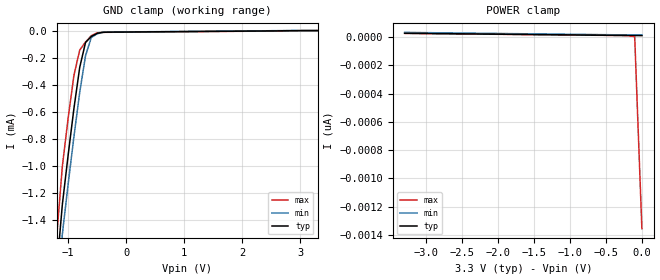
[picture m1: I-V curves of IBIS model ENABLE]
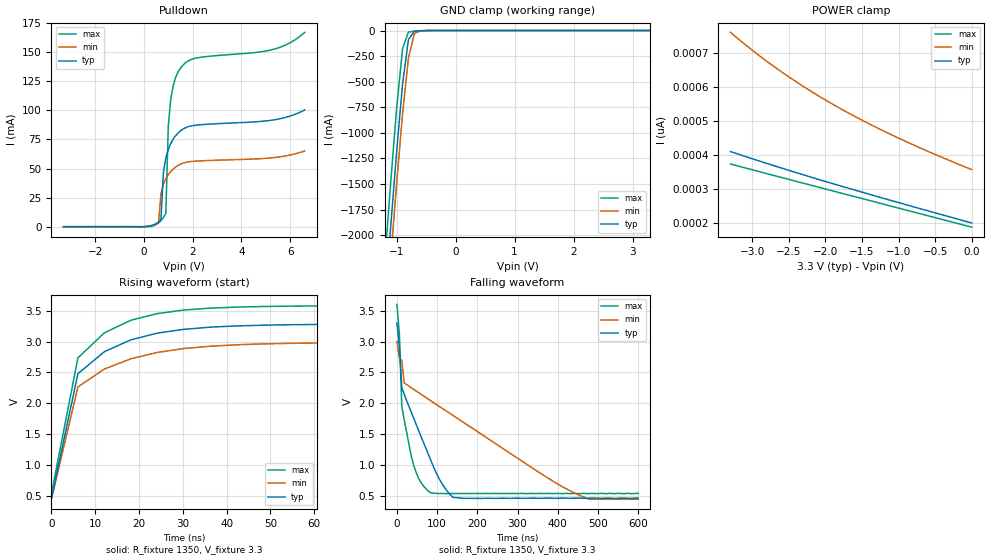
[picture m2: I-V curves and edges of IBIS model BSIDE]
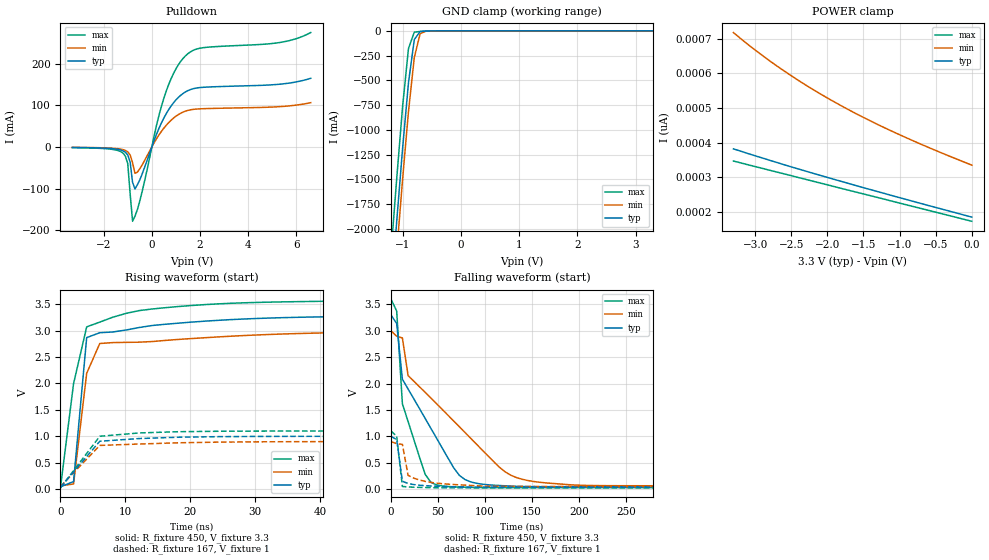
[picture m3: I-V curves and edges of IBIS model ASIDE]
| PCA9508 IBIS Model
[IBIS Ver]   4.0
[Comment Char]   |_char
| vdd: nom:3.3v, min:3v, max:3.6v
[File name]   pca9508.ibs
[File Rev]   2
[Date]   September 14, 2009 4:38:58 PM
[Source]
Generated by Nipun Chaplot at NXP Tempe using IBIS Toolkit
[Notes]
|The package model information is simulated at 400 kHz,
|which is the maximum system operating frequency.
[Disclaimer]
(C) Copyright 2007 NXP Semiconductors
All rights reserved
NXP Semiconductors (NXP) does not warrant that this model and any other
accompanying information (Model) accurately or fully represents the
operating characteristics and specifications of the semiconductor
products to which the Model relates.  Moreover, the Model is furnished
on an "as is" and with "all faults" basis, and without support or
warranty of any kind.  NXP disclaims all warranties, whether expressed
or implied or statutory, including without limitation all implied
warranties of non-infringement, merchantability and fitness for any
purpose, and those arising from a course of dealing or usage of trade.
NXP does not convey any license under its or any third party's patents,
copyrights or other intellectual property or proprietary rights.
You and your company assume any and all risks and liability arising out
of the application or use of the Model.
In no event shall NXP be liable for any direct, indirect, special,
consequential or incidental damages, however caused, whether in
warranty, contract or tort (including negligence), strict liability or
other legal theory, including, without limitation, for lost profits,
business interruption, or corruption or loss of data or information,
arising out of or in connection with the use of or the inability to use
the Model, even if NXP has been advised of the possibility of such
damages.
NXP provides the Model as a courtesy to our customers. You and your
company shall not distribute, convey, sell, or give the Model to anyone
else without receiving prior written permission from NXP.
NXP reserves the right to make changes without notice to the Model to
improve reliability, function, or design.
Please be aware that your receipt and subsequent use of the Model shall
serve as acceptance of these terms and conditions.  If you do not
accept these terms, return or destroy the Model immediately.
[Copyright]
(C) Copyright 2009 NXP Semiconductors  All rights reserved
| TSSOP8 Package
[Component]   PCA9508DP
Si_location Die
Timing_location Pin
[Manufacturer]   NXP Semiconductors
[Package]
|Simulation frequency: 100MHz
|variable   typ   min   max
R_pkg   33.7m   30.1m   37.3m
L_pkg   1.74n   1.67n   1.81n
C_pkg   0.428p   0.422p   0.434p
[Pin] signal_name   model_name   R_pin   L_pin   C_pin
1   VCCA   POWER   5.47E-02  2.21E-09  4.81E-13
2   SCLA   ASIDE   4.14E-02  1.54E-09  4.20E-13
3   SDAA   ASIDE   4.14E-02  1.55E-09  4.20E-13
4   GND   GND   5.47E-02  2.21E-09  4.80E-13
5   EN   ENABLE   5.47E-02  2.21E-09  4.78E-13
6   SDAB   BSIDE   4.14E-02  1.55E-09  4.17E-13
7   SCLB   BSIDE   4.14E-02  1.54E-09  4.17E-13
8   VCCB   POWER   5.47E-02  2.21E-09  4.79E-13
[Package Model]   tssop8_sot505EC12
|The package model information is simulated at 400 kHz,
|which is the maximum system operating frequency.
| SO-8 package
[Component]   PCA9508D
Si_location Die
Timing_location Pin
[Manufacturer]   NXP Semiconductors
[Package]
|Simulation frequency: 100MHz
|variable   typ   min   max
R_pkg   4.81E-02   4.14E-02   5.47E-02
L_pkg   1.88E-09   1.54E-09   2.21E-09
C_pkg   0.449E-12   0.417E-12   0.481E-12
[Pin] signal_name   model_name   R_pin   L_pin   C_pin
1   VCCA   POWER   37.3m   1.81nH   0.428pF
2   SCLA   ASIDE   30.1m   1.67nH   0.422pF
3   SDAA   ASIDE   30.1m   1.67nH   0.428pF
4   GND   GND   37.3m   1.81nH   0.434pF
5   EN   ENABLE   37.3m   1.81nH   0.428pF
6   SDAB   BSIDE   30.1m   1.67nH   0.422pF
7   SCLB   BSIDE   30.1m   1.67nH   0.428pF
8   VCCB   POWER   37.3m   1.81nH   0.434pF
[Package Model]   so8_sot96bl53
|   PACKAGE MODEL SO-8
[Define Package Model]  so8_sot96bl53
[Manufacturer]  NXP
[OEM]   NXP Semiconductors
[Description]   Full package IBIS model.Simulated @ 400kHz
[Number Of Pins]  8
[Pin Numbers]
|Pin Num   Terminal Name
1   | Lead1:pin1
2   | Lead2:pin2
3   | Lead3:pin3
4   | Lead4:pin4
5   | Lead5:pin5
6   | Lead6:pin6
7   | Lead7:pin7
8   | Lead8:pin8
[Model Data]
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[End Model Data]
[End Package Model]
|   PACKAGE MODEL TSSOP8
[Define Package Model]  tssop8_sot505EC12
[Manufacturer]  NXP
[OEM]   NXP Semiconductors
[Description]   Full package IBIS model. Simulated @ 400kHz
[Number Of Pins]  8
[Pin Numbers]
|Pin Num   Terminal Name
1   | Lead1:pin1
2   | Lead2:pin2
3   | Lead3:pin3
4   | Lead4:pin4
5   | Lead5:pin5
6   | Lead6:pin6
7   | Lead7:pin7
8   | Lead8:pin8
[Model Data]
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[End Model Data]
[End Package Model]
| Models and submodels in the file (3): ENABLE (Input), BSIDE (I/O_open_drain), ASIDE (I/O_open_drain)
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|The package model information is simulated at 400 kHz,
|which is the maximum system operating frequency.
[Model]   ENABLE
Model_type Input
Vinh=2.31
Vinl=0.99
|Subparameter   typ   min   max
C_comp   1.86p   1.7p   2p
[Model Spec]
Vinh   2.31   1.89   5.5
Vinl   0.99   0.40   1.65
[Temperature Range] 27   85   -40
[Voltage Range]   3.3   3   3.6
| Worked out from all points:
|   GND clamp passes 1 mA (typ) near -1.02 V on its own axis
[GND Clamp]
-3.3V     -17.95A    -17.36A    -18.67A
-1.2V     -1.789mA   -2.001mA   -1.542mA
-1.1V     -1.289mA   -1.508mA   -1.007mA
-1V       -922.8uA   -1.138mA   -649.1uA
-900mV    -576.7uA   -785.3uA   -331.4uA
-800mV    -272.4uA   -456.9uA   -144.1uA
-700mV    -88.06uA   -186.1uA   -84.85uA
-600mV    -43.6uA    -50.75uA   -37.68uA
-500mV    -20.3uA    -24.22uA   -16.64uA
-300mV    -11.67uA   -10.77uA   -12.63uA
3.3V      9.969pA    13.77pA    -1.356nA
[POWER Clamp]
-3.3V     26.62pA    32.76pA    25.82pA
-200mV    11.03pA    14.89pA    10.27pA
-100mV    10.53pA    14.32pA    2.629pA
0V        9.962pA    13.77pA    -1.356nA
[Model]   BSIDE
Model_type I/O_open_drain
Vinh=2.31
Vinl=0.99
Vref=3.3
Vmeas=0.65
Rref=1350
Cref=50p
|Subparameter   typ   min   max
C_comp   4.28p   4.1p   4.4p
[Model Spec]
Vinh   2.31   1.89   5.5
Vinl   0.99   0.40   1.65
Vmeas   1.65   1.35   2.75
[Temperature Range] 27   85   -40
[Voltage Range]   3.3   3   3.6
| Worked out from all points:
|   slope of the pulldown table from 0 to 0.495 V, typ, clamps not added: 200 ohm
|   GND clamp passes 1 mA (typ) near -0.52 V on its own axis
|   falling waveform, R_fixture 1350, V_fixture 3.3: 20-80 % time 79.4ns typ, 320ns min, 28.8ns max; typ from 3.3 V to 0.464 V
|   rising waveform, R_fixture 1350, V_fixture 3.3: 20-80 % time 8.61ns typ, 8.99ns min, 8.11ns max; typ from 0.463 V to 3.3 V
[Pulldown]
-3.3V     0A         0A         0A
600mV     3.943mA    3.455mA    3.206mA
700mV     6.084mA    27.99mA    5.214mA
800mV     46.34mA    36.75mA    7.871mA
900mV     59.04mA    41.34mA    11.66mA
1V        66.35mA    44.71mA    86.27mA
1.1V      71.51mA    47.35mA    109.2mA
1.3V      78.18mA    51.26mA    128.3mA
1.5V      82.38mA    53.79mA    136.3mA
2.2V      87.4mA     56.44mA    145.2mA
5.4V      92.07mA    59.57mA    153mA
6.6V      100.4mA    65.12mA    167.1mA
[GND Clamp]
-3.3V     -37.68A    -37.34A    -38.04A
-1.2V     -2.671A    -2.981A    -2.242A
-1.1V     -1.91A     -2.223A    -1.478A
-1V       -1.181A    -1.492A    -758.7mA
-900mV    -524.4mA   -815.2mA   -178.8mA
-800mV    -88.63mA   -269.5mA   -14.24mA
-700mV    -7.072mA   -29.66mA   -6.721mA
-600mV    -2.61mA    -3.048mA   -2.176mA
3.3V      200.1pA    356.8pA    187.8pA
[POWER Clamp]
-3.3V     410pA      760.5pA    373.4pA
-2.9V     381.9pA    691pA      350.8pA
-2.6V     361.6pA    644.2pA    333.8pA
-2.2V     335pA      587.6pA    311.2pA
-1.8V     309.4pA    536.8pA    288.7pA
-1.3V     278.3pA    480.4pA    260.7pA
-900mV    253.9pA    439.5pA    238.2pA
0V        200.1pA    356.8pA    187.8pA
[Falling Waveform]
R_fixture=1350
V_fixture=3.3
V_fixture_min=3
V_fixture_max=3.6
0s        3.3V       3V         3.6V
6.061ns   2.917V     2.739V     3.13V
12.12ns   2.252V     2.693V     1.951V
18.18ns   2.149V     2.326V     1.729V
42.42ns   1.749V     2.222V     978.8mV
78.79ns   1.165V     2.064V     571.2mV
109.1ns   731.6mV    1.933V     538.9mV
139.4ns   475.2mV    1.803V     538.5mV
454.5ns   463.7mV    508.8mV    537.1mV
600ns     464.1mV    448mV      540.8mV
[Rising Waveform]
R_fixture=1350
V_fixture=3.3
V_fixture_min=3
V_fixture_max=3.6
0s        462.9mV    449.4mV    539.4mV
6.061ns   2.482V     2.267V     2.737V
12.12ns   2.837V     2.557V     3.143V
18.18ns   3.029V     2.722V     3.345V
24.24ns   3.137V     2.825V     3.453V
30.3ns    3.198V     2.888V     3.51V
36.36ns   3.233V     2.925V     3.541V
48.48ns   3.265V     2.962V     3.567V
84.85ns   3.284V     2.986V     3.582V
600ns     3.299V     2.998V     3.599V
[Ramp]
R_load=1350
dV/dt_r   4.966E-3/1.215E-8   2.879E-3/1.635E-8   7.929E-3/7.340E-9
dV/dt_f   1.702E+0/7.706E-8   1.531E+0/3.202E-7   1.836E+0/2.904E-8
|[End   BSIDE
[Model]   ASIDE
Model_type I/O_open_drain
Vinh=2.31
Vinl=0.99
Vref=3.3
Vmeas=0.65
Rref=450
Cref=50p
|Subparameter   typ   min   max
C_comp   3.97p   3.8p   4.1p
[Model Spec]
Vinh   2.31   0.63   5.5
Vinl   0.99   0.27   1.65
Vmeas   0.99   0.27   1.65
[Temperature Range] 27   85   -40
[Voltage Range]   3.3   3   3.6
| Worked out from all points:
|   slope of the pulldown table from 0 to 0.495 V, typ, clamps not added: 7.18 ohm
|   GND clamp passes 1 mA (typ) near -0.52 V on its own axis
|   falling waveform, R_fixture 450, V_fixture 3.3: 20-80 % time 48.3ns typ, 86ns min, 20.1ns max; typ from 3.3 V to 0.044 V
|   falling waveform, R_fixture 167, V_fixture 1: 20-80 % time 4.46ns typ, 9.58ns min, 4.11ns max; typ from 1 V to 0.035 V
|   rising waveform, R_fixture 450, V_fixture 3.3: 20-80 % time 1.45ns typ, 2.27ns min, 2.95ns max; typ from 0.043 V to 3.3 V
|   rising waveform, R_fixture 167, V_fixture 1: 20-80 % time 4.03ns typ, 3.98ns min, 4.01ns max; typ from 0.035 V to 1 V
[Pulldown]
-3.3V     -1.37mA    -1.08mA    -1.78mA
-1.2V     -9.287mA   -6.495mA   -14.72mA
-1V       -19.25mA   -11.89mA   -40.21mA
-900mV    -36.58mA   -19.24mA   -112.9mA
-800mV    -85.08mA   -38.24mA   -178.8mA
-700mV    -101.1mA   -63.27mA   -166.5mA
-600mV    -91mA      -60.81mA   -150.6mA
500mV     69.44mA    45.13mA    117mA
900mV     106mA      69.26mA    176.4mA
1.4V      132.3mA    86.05mA    219mA
2V        142.6mA    91.51mA    237.3mA
6.6V      164.9mA    106.3mA    274.8mA
[GND Clamp]
-3.3V     -37.68A    -37.34A    -38.04A
-1.2V     -2.671A    -2.981A    -2.242A
-1.1V     -1.91A     -2.223A    -1.478A
-1V       -1.181A    -1.492A    -758.5mA
-900mV    -524.1mA   -815mA     -178.5mA
-800mV    -88.25mA   -269.1mA   -13.8mA
-700mV    -6.842mA   -29.34mA   -6.41mA
-600mV    -2.483mA   -2.935mA   -2.068mA
3.3V      185.4pA    335.3pA    173.4pA
[POWER Clamp]
-3.3V     382.2pA    717.4pA    347pA
-3V       362.2pA    667.1pA    331.2pA
-2.6V     336.6pA    607pA      310.2pA
-2.2V     312pA      553.4pA    289pA
-1.8V     288pA      505.5pA    267.9pA
-1.3V     258.8pA    452.1pA    241.7pA
-1V       241.5pA    422.9pA    225.8pA
-500mV    213.3pA    377.6pA    199.6pA
0V        185.4pA    335.3pA    173.4pA
[Falling Waveform]
R_fixture=450
V_fixture=3.3
V_fixture_min=3
V_fixture_max=3.6
0s        3.3V       3V         3.6V
6.061ns   3.137V     2.896V     3.374V
12.12ns   2.082V     2.864V     1.617V
18.18ns   1.896V     2.151V     1.28V
36.36ns   1.338V     1.832V     279.6mV
48.48ns   963.1mV    1.617V     77.99mV
78.79ns   179.2mV    1.071V     35.55mV
121.2ns   62.41mV    327.7mV    28.42mV
151.5ns   46.21mV    144.1mV    28.23mV
600ns     44.04mV    62.24mV    28.14mV
[Falling Waveform]
R_fixture=167
V_fixture=1
V_fixture_min=0.9
V_fixture_max=1.1
0s        1V         900mV      1.1V
6.061ns   936mV      860.2mV    1.003V
12.12ns   148.4mV    846.9mV    49.72mV
18.18ns   105.1mV    260.1mV    40.3mV
24.24ns   85.33mV    207.1mV    35.22mV
36.36ns   64.21mV    145.7mV    29.46mV
60.61ns   45.37mV    93.13mV    23.67mV
96.97ns   35.98mV    58.01mV    23.02mV
127.3ns   35.39mV    50.32mV    22.95mV
600ns     35.12mV    48.44mV    22.9mV
[Rising Waveform]
R_fixture=450
V_fixture=3.3
V_fixture_min=3
V_fixture_max=3.6
0s        43.1mV     61.36mV    27.03mV
2.02ns    142.9mV    96.25mV    1.996V
4.04ns    2.869V     2.192V     3.072V
6.061ns   2.961V     2.757V     3.162V
8.081ns   2.975V     2.774V     3.255V
12.12ns   3.06V      2.782V     3.38V
16.16ns   3.121V     2.815V     3.435V
26.26ns   3.209V     2.895V     3.519V
44.44ns   3.268V     2.966V     3.562V
200ns     3.298V     2.997V     3.596V
[Rising Waveform]
R_fixture=167
V_fixture=1
V_fixture_min=0.9
V_fixture_max=1.1
0s        35.1mV     48.4mV     22.9mV
6.061ns   905.7mV    826.7mV    1V
12.12ns   956.8mV    853.1mV    1.063V
18.18ns   981.9mV    876.5mV    1.086V
30.3ns    996.9mV    894.8mV    1.098V
54.55ns   999.7mV    899.7mV    1.099V
600ns     999.9mV    899.9mV    1.1V
[Ramp]
R_load=167
dV/dt_r   5.173E-6/1.058E-8   1.778E-6/1.483E-8   1.431E-5/7.092E-9
dV/dt_f   4.551E-3/9.066E-9   4.450E-3/1.346E-8   3.972E-3/5.680E-9
|[End   ASIDE
